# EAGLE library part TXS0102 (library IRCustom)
2-Bit Bi-Directional Level Shifter (I2C, etc.) Designed for I2C devices and has internal pullups. Not to be confused with TXB010x series. 1.2V-3.6V (VCCA) to 1.65V-5.5V (VCCB) bi-directional level shifter with auto direction sensing. Max data rate - 24Mbps (Push Pull), 2Mbps (Open Drain) Digikey: 296-21931-1-ND
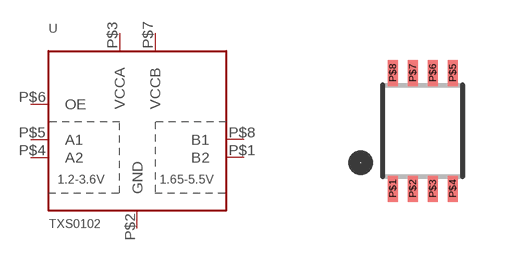
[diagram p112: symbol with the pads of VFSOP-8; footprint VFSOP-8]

Designator prefix U

## TXS0102  [VFSOP-8]
P$1  B2
P$2  GND
P$3  VCCA
P$4  A2
P$5  A1
P$6  OE
P$7  VCCB
P$8  B1

## Footprint VFSOP-8 (pad centres in mm)
VFSOP8 - 0.5mm pitch, 2.0x2.3mm Source: http://focus.ti.com/lit/ds/symlink/txs0102.pdf
smd 0.25 x 0.65: P$1 -0.75,-1.45; P$2 -0.25,-1.45; P$3 0.25,-1.45; P$4 0.75,-1.45; P$5 0.75,1.45; P$6 0.25,1.45; P$7 -0.25,1.45; P$8 -0.75,1.45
